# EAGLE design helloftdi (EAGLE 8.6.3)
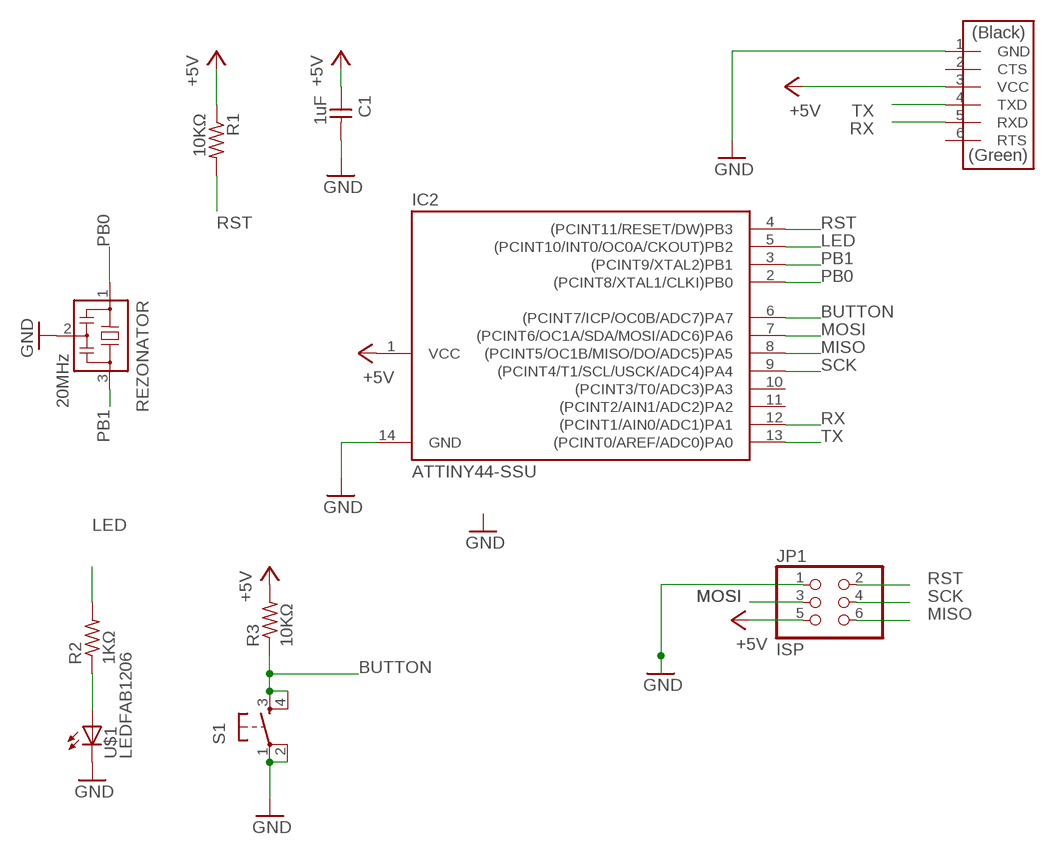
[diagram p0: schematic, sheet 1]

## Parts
C1  1uF  CAP-UNPOLARIZEDFAB  [C1206FAB]
IC2  ATTINY44-SSU  [SOIC14]
JP1  ISP  PINHD-2X3-SMD  [2X03SMD]
R1  10KΩ  RES-US1206FAB  [R1206FAB]
R2  1KΩ  RES-US1206FAB  [R1206FAB]
R3  10KΩ  RES-US1206FAB  [R1206FAB]
REZONATOR  20MHz  RESONATOR  [EFOBM]
S1  6MM_SWITCH6MM_SWITCH  [6MM_SWITCH]
U$1  LEDFAB1206  [LED1206FAB]
U$2  FTDI-SMD-HEADER  [1X06SMD]

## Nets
+5V: C1.1 IC2.1(VCC) JP1.5 R1.1 R3.2 U$2.3(VCC)
BUTTON: IC2.6((PCINT7/ICP/OC0B/ADC7)PA7) R3.1 S1.3(S) S1.4(S1)
GND: C1.2 IC2.14(GND) JP1.1 REZONATOR.2 S1.1(P) S1.2(P1) U$1.2(C) U$2.1(GND)
LED: IC2.5((PCINT10/INT0/OC0A/CKOUT)PB2) R2.2
MISO: IC2.8((PCINT5/OC1B/MISO/DO/ADC5)PA5) JP1.6
MOSI: IC2.7((PCINT6/OC1A/SDA/MOSI/ADC6)PA6) JP1.3
N$1: R2.1 U$1.1(A)
PB0: IC2.2((PCINT8/XTAL1/CLKI)PB0) REZONATOR.1
PB1: IC2.3((PCINT9/XTAL2)PB1) REZONATOR.3
RST: IC2.4((PCINT11/RESET/DW)PB3) JP1.2 R1.2
RX: IC2.12((PCINT1/AIN0/ADC1)PA1) U$2.5(RXD)
SCK: IC2.9((PCINT4/T1/SCL/USCK/ADC4)PA4) JP1.4
TX: IC2.13((PCINT0/AREF/ADC0)PA0) U$2.4(TXD)
Unconnected: IC2.10((PCINT3/T0/ADC3)PA3) IC2.11((PCINT2/AIN1/ADC2)PA2) U$2.2(CTS) U$2.6(RTS)

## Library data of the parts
C1 = fab:CAP-UNPOLARIZED
IC2 = fab:ATTINY44
JP1 = fab:PINHD-2X3-SMD: PIN HEADER
R1 R2 = fab:RES-US: Resistor (US Symbol)
R3 = HelloKamakura:RES-US: Resistor (US Symbol)
REZONATOR = fab:RESONATOR
S1 = fab:6MM_SWITCH: OMRON SWITCH
U$1 = fab:LED: LED
U$2 = fab:FTDI-SMD-HEADER

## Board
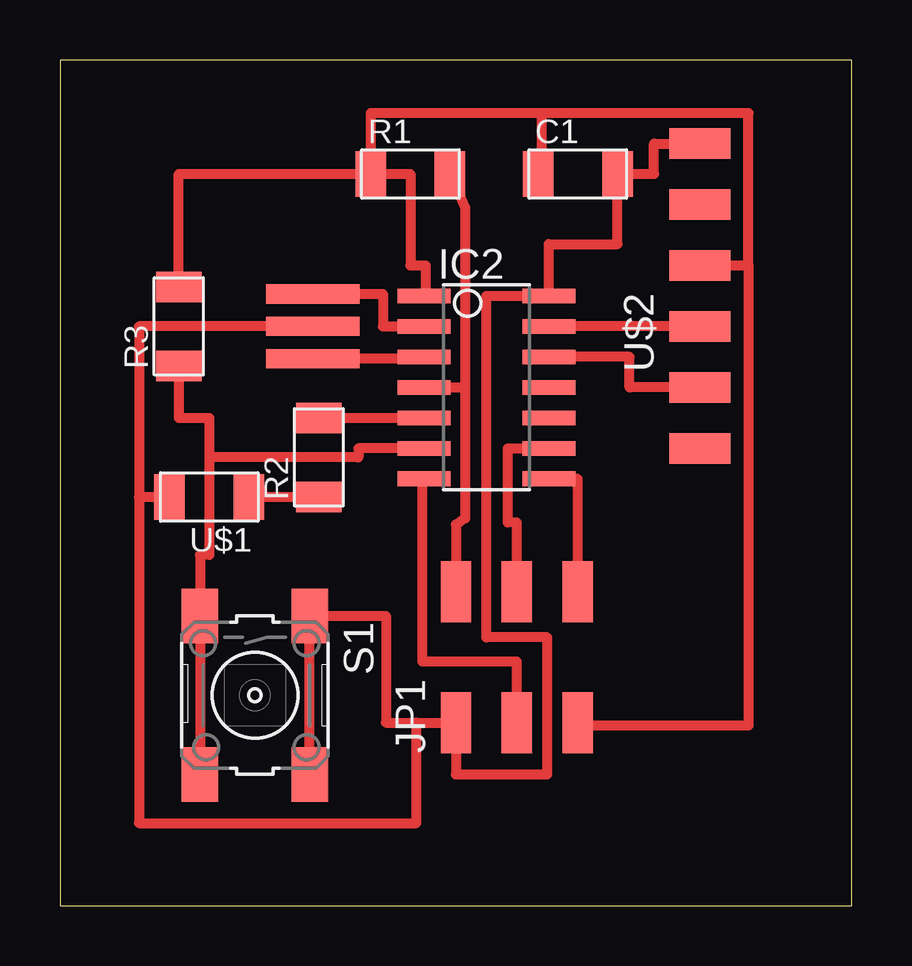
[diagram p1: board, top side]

Size 33 x 35.23 mm. Coordinates in mm from the lower left corner, seen from the top.
Outline: 0,0 33,0 33,35.23 0,35.23 0,0
Copper layers (1*16): Top 0.035mm / dielectric 1.5mm / Bottom 0.035mm
Design rules "default *": minimum track width 6mil, minimum drill 0.35mm, track to track 0.4mm, track to pad 0.4mm, pad to pad 0.4mm, via to via 0.4mm, smd to smd 0.4mm, copper to edge 40mil, drill to drill 6mil, minimum pad ring 10mil, minimum via ring 8mil, stop-mask expansion 4mil, vias tented up to drill 0mil, thermal gap 10mil

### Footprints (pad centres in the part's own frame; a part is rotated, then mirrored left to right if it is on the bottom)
C1206FAB = smd 1.27 x 1.905: 1 -1.651,0; 2 1.651,0
SOIC14 = smd 0.61 x 2.21: 1 -3.81,-2.603; 2 -2.54,-2.603; 3 -1.27,-2.603; 4 0,-2.603; 5 1.27,-2.603; 6 2.54,-2.603; 7 3.81,-2.603; 8 3.81,2.603; 9 2.54,2.603; 10 1.27,2.603; 11 0,2.603; 12 -1.27,2.603; 13 -2.54,2.603; 14 -3.81,2.603
2X03SMD = smd 2.54 x 1.27: 1 -2.54,2.54; 2 2.92,2.54; 3 -2.54,0; 4 2.92,0; 5 -2.54,-2.54; 6 2.92,-2.54
R1206FAB = smd 1.27 x 1.905: 1 -1.651,0; 2 1.651,0
EFOBM = smd 0.8 x 3.9: 1 -1.35,0; 2 0,0; 3 1.35,0
6MM_SWITCH = smd 2.286 x 1.524: 1 -3.302,2.286; 2 3.302,2.286; 3 -3.302,-2.286; 4 3.302,-2.286
LED1206FAB = smd 1.27 x 1.905: 1 -1.651,0; 2 1.651,0
1X06SMD = smd 2.54 x 1.27: 1 0,6.35; 2 0,3.81; 3 0,1.27; 4 0,-1.27; 5 0,-3.81; 6 0,-6.35

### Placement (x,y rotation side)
C1  21.59,30.48 0 top
IC2  17.78,21.59 270 top
JP1  19.05,10.16 90 top
R1  14.61,30.48 0 top
R2  10.79,18.67 90 top
R3  4.95,24.13 90 top
REZONATOR  10.54,24.13 270 top
S1  8.13,8.76 270 top
U$1  6.22,17.02 180 top
U$2  26.67,25.4 0 top

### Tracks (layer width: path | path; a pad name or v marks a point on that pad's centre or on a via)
+5V
  Top 0.406: R1.1 14.61,30.48 14.61,26.67 15.24,26.67 15.24,25.4 IC2.1 | U$2.3 28.7,26.67 | 28.7,26.67 28.7,33.02 20.07,33.02 | 20.07,33.02 20.07,30.48 C1.1 | 20.07,33.02 12.95,33.02 R1.1 | 28.7,26.67 28.7,7.49 21.59,7.49 JP1.5 | R3.2 4.95,30.48 R1.1
BUTTON
  Top 0.406: 5.84,22.48 R3.1 4.95,20.32 6.22,20.32 6.22,18.67 | S1.4 S1.3 5.84,14.61 6.22,14.61 6.22,18.67 | IC2.6 12.45,19.05 12.45,18.67 6.22,18.67
GND
  Top 0.406: U$2.1 24.77,31.75 24.77,30.48 C1.2 23.24,27.56 20.38,27.56 IC2.14 17.78,25.4 17.78,11.18 20.32,11.18 20.32,5.46 16.51,5.46 JP1.1 14.86,7.62 | REZONATOR.2 3.3,24.13 3.3,17.02 | 3.3,17.02 3.3,3.43 14.86,3.43 14.86,7.62 | 14.86,7.62 13.59,7.62 13.59,12.06 S1.1 S1.2 | U$1.2 3.3,17.02
LED
  Top 0.406: R2.2 IC2.5
MISO
  Top 0.406: JP1.6 21.59,17.78 IC2.8
MOSI
  Top 0.406: JP1.3 19.05,10.16 15.11,10.16 15.11,17.78 IC2.7
N$1
  Top 0.406: R2.1 U$1.1
PB0
  Top 0.406: REZONATOR.1 13.46,25.48 13.46,24.13 IC2.2
PB1
  Top 0.406: IC2.3 15.18,22.78 REZONATOR.3
RST
  Top 0.406: R1.2 16.89,29.08 16.89,21.59 | JP1.2 16.51,15.88 16.89,16.13 16.89,21.59 | IC2.4 16.89,21.59
RX
  Top 0.406: U$2.5 23.75,21.59 23.75,22.86 IC2.12
SCK
  Top 0.406: JP1.4 19.05,15.96 18.68,15.96 18.68,17.65 18.67,18.92 18.67,19.05 IC2.9
TX
  Top 0.406: U$2.4 IC2.13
